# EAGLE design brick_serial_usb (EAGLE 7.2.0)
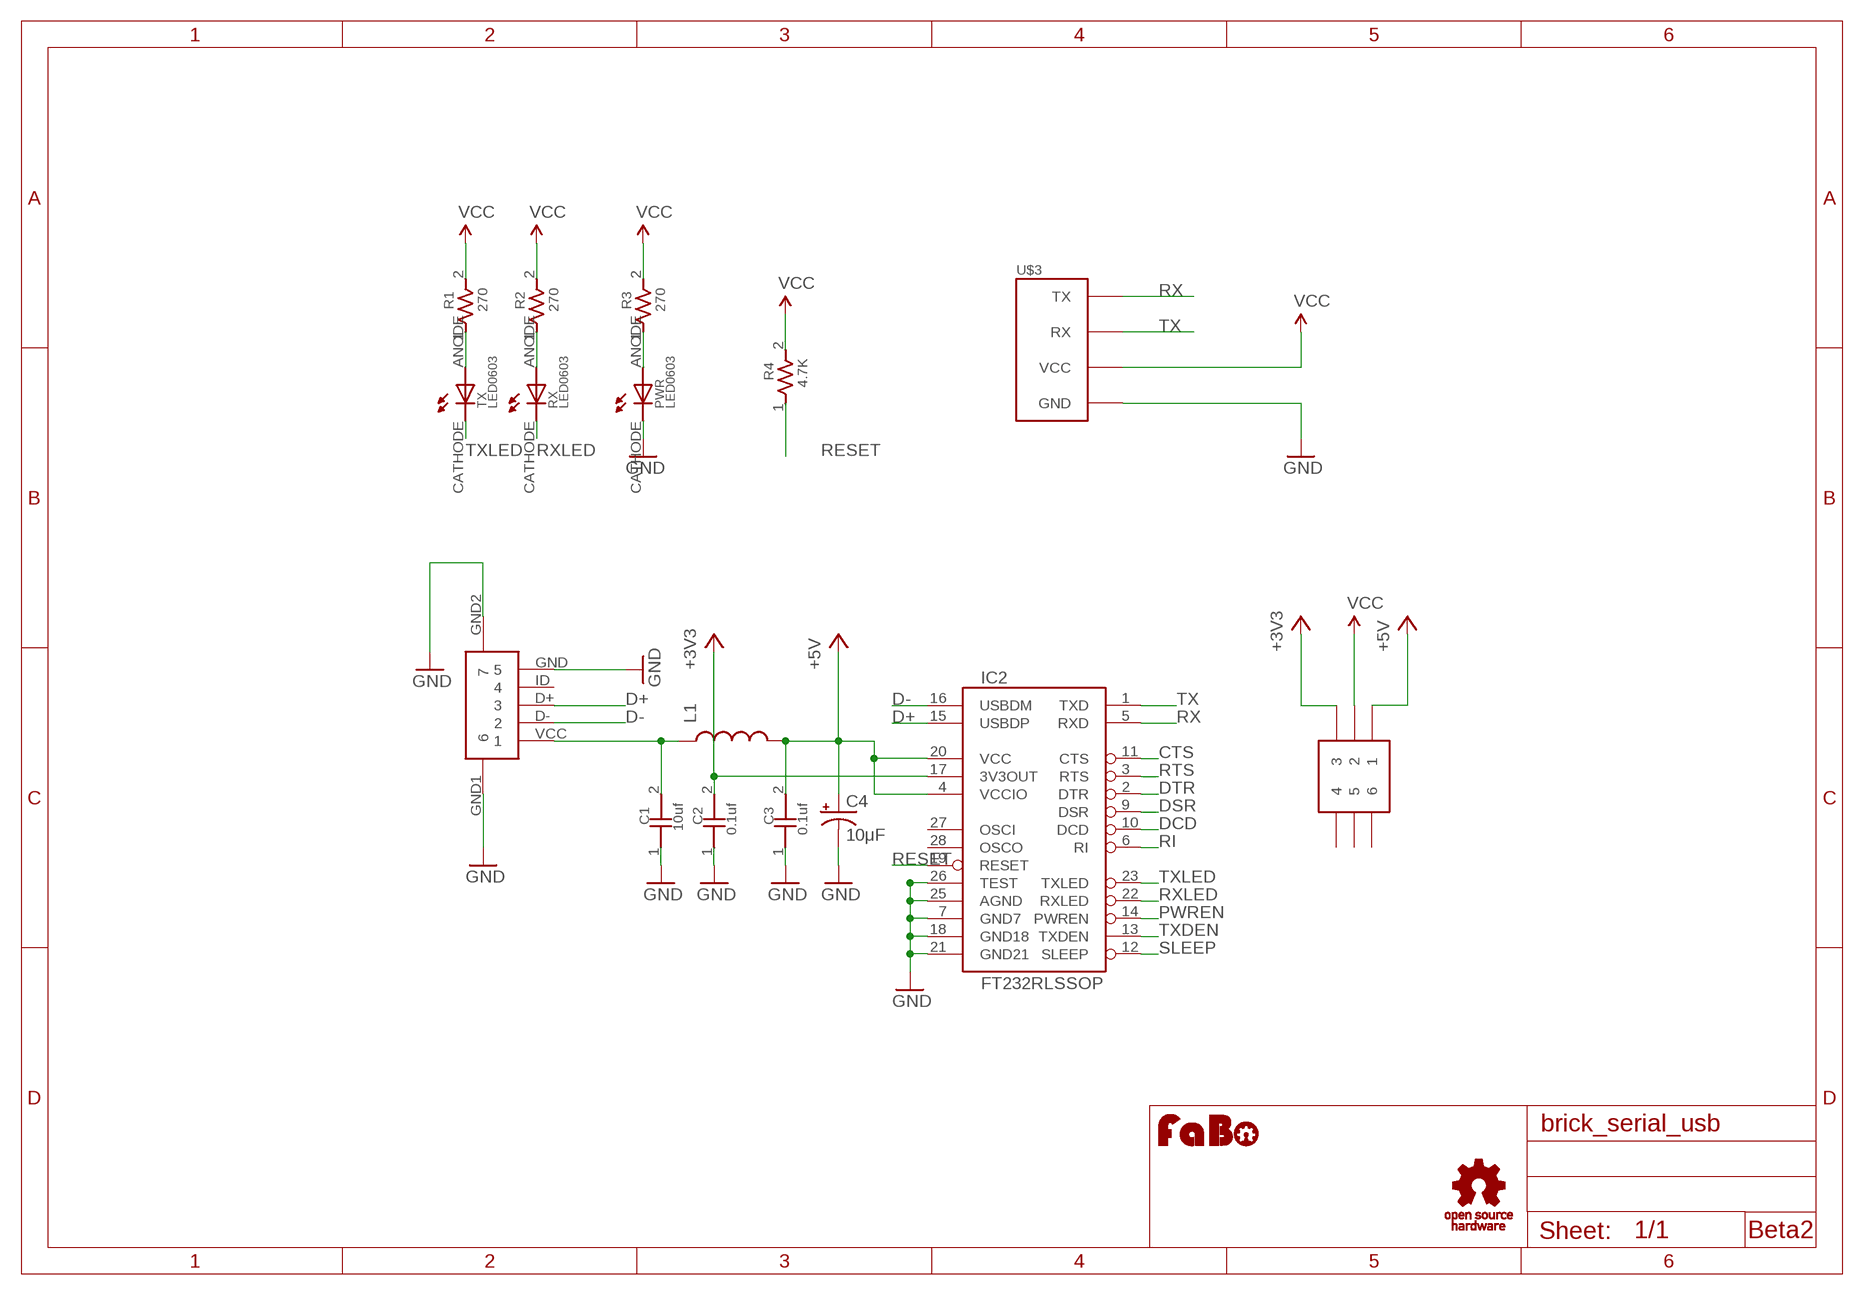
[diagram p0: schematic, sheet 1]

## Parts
C1  10uf  CAPACITOR0603  [0603]
C2  0.1uf  CAPACITOR0603  [0603]
C3  0.1uf  CAPACITOR0603  [0603]
C4  10μF  CAP_POL1206  [EIA3216]
IC2  FT232RLSSOP  [SSOP28DB]
L1  INDUCTOR0603  [0603]
PWR  LED0603  [0603]
R1  270  RESISTOR0603  [0603]
R2  270  RESISTOR0603  [0603]
R3  270  RESISTOR0603  [0603]
R4  4.7K  RESISTOR0603  [0603]
RX  LED0603  [0603]
TX  LED0603  [0603]
U$1  USB-MICRO-B-FEMALE  [USB-MICRO-B-FEMALE]
U$2  C&K_JS202011SCQN  [C&K_JS202011SCQN]
U$3  BRICK_SERIAL  [BRICK_SERIAL]
U$5  LOGO_OSHW_T-S  [LOGO_OSHW_T_S]
U$6  LOGO_FABO-S  [LOGO_FABO_S]

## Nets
+3V3: C2.2 IC2.17(3V3OUT) U$2.3
+5V: C3.2 C4.A(+) IC2.4(VCCIO) IC2.20(VCC) L1.2 U$2.1
CTS: IC2.11(CTS)
D+: IC2.15(USBDP) U$1.D+
D-: IC2.16(USBDM) U$1.D-
DCD: IC2.10(DCD)
DSR: IC2.9(DSR)
DTR: IC2.2(DTR)
GND: C1.1 C2.1 C3.1 C4.C(-) IC2.7(GND7) IC2.18(GND18) IC2.21(GND21) IC2.25(AGND) IC2.26(TEST) PWR.CATHODE U$1.GND U$1.GND1 U$1.GND2 U$3.GND
N$1: C1.2 L1.1 U$1.VCC
N$2: R1.1 TX.ANODE
N$5: R2.1 RX.ANODE
N$6: PWR.ANODE R3.1
PWREN: IC2.14(PWREN)
RESET: IC2.19(RESET) R4.1
RI: IC2.6(RI)
RTS: IC2.3(RTS)
RX: IC2.5(RXD) U$3.TX
RXLED: IC2.22(RXLED) RX.CATHODE
SLEEP: IC2.12(SLEEP)
TX: IC2.1(TXD) U$3.RX
TXDEN: IC2.13(TXDEN)
TXLED: IC2.23(TXLED) TX.CATHODE
VCC: R1.2 R2.2 R3.2 R4.2 U$2.2 U$3.VCC
Unconnected: IC2.27(OSCI) IC2.28(OSCO) U$1.ID U$2.4 U$2.5 U$2.6

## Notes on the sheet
- Beta2

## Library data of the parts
C1-C3 = GClue-Capacitor:CAPACITOR
C4 = SparkFun:CAP_POL: Capacitor Polarized
IC2 = SparkFun:FT232RL: USB UART FT232RL 4th Generation USB UART (USB <-> Serial) Controller. Spark Fun Electronics SKU : COM-00650
L1 = SparkFun:INDUCTOR: Inductors
PWR RX TX = GClue-LED:LED
R1-R4 = GClue-Resistors:RESISTOR
U$1 = gclue:USB-MICRO-B-FEMALE
U$2 = gclueParts:C&K_JS202011SCQN
U$3 = gclue:BRICK_SERIAL: FaBo Brick 4pin(SERIAL)
U$5 = gclue:LOGO_OSHW_T
U$6 = FaBo:LOGO_FABO

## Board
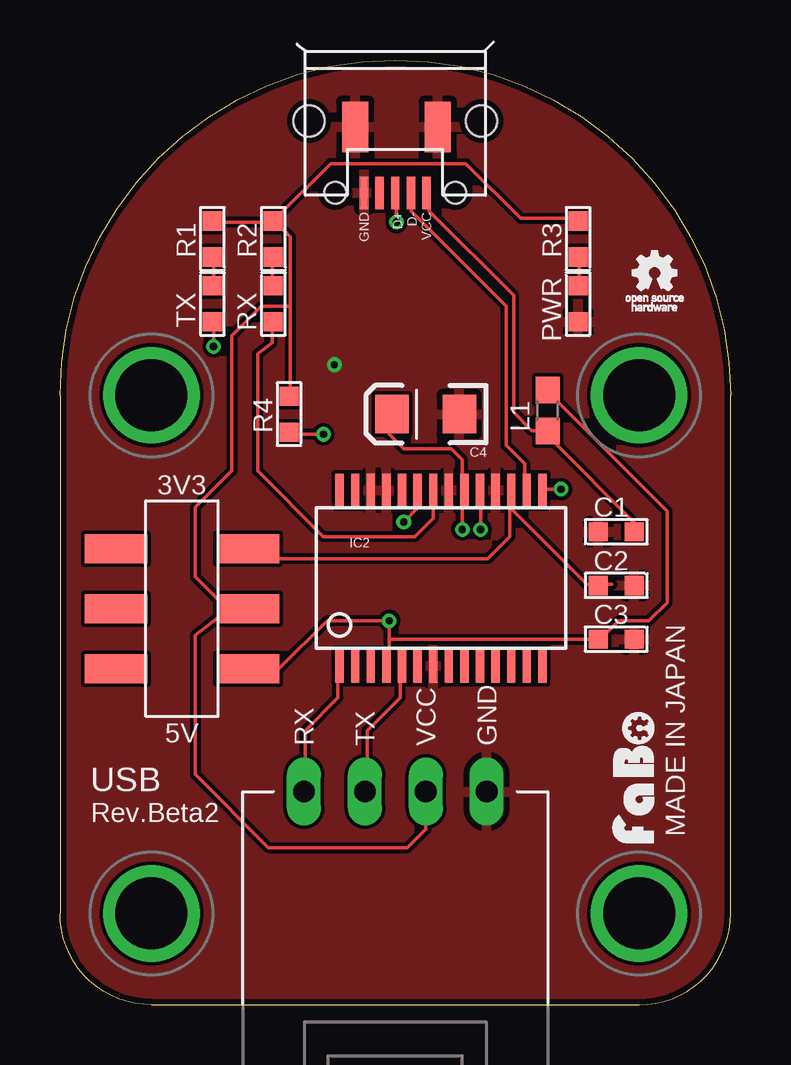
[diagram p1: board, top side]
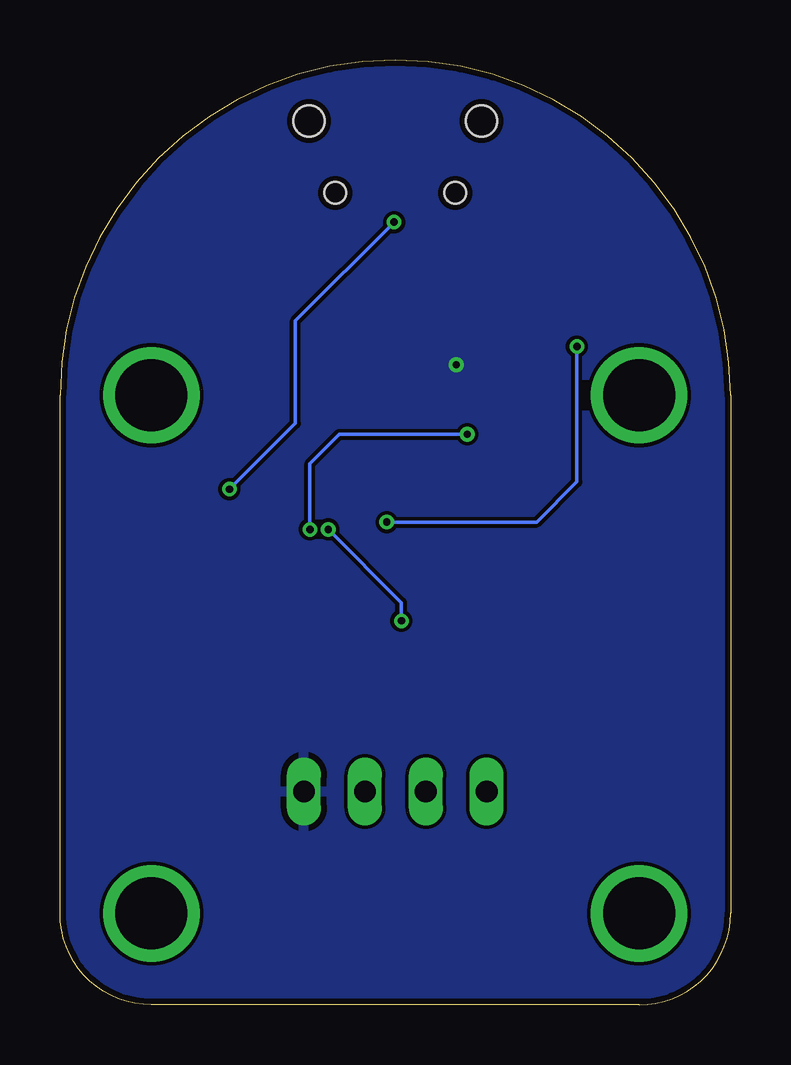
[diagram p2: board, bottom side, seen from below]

Size 27.94 x 39.37 mm. Coordinates in mm from the lower left corner, seen from the top.
Copper layers (1*16): Top 0.035mm / dielectric 1.5mm / Bottom 0.035mm
Design rules "Elecrow_2-layer_eagle_rule": minimum track width 6mil, minimum drill 12mil, track to track 6mil, track to pad 6mil, pad to pad 6mil, via to via 6mil, smd to smd 0mil, copper to edge 10mil, drill to drill 10mil, minimum pad ring 10mil, minimum via ring 6mil, stop-mask expansion 2mil, vias tented up to drill 100mil, thermal gap 10mil

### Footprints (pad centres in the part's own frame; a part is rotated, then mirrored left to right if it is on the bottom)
0603 = smd 0.8 x 0.8: 1 -0.75,0; 2 0.75,0
EIA3216 = smd 1.4 x 1.6: A 1.4,0; C -1.4,0
SSOP28DB = smd 0.348 x 1.397: 1 -4.225,-3.656; 2 -3.575,-3.656; 3 -2.925,-3.656; 4 -2.275,-3.656; 5 -1.625,-3.656; 6 -0.975,-3.656; 7 -0.325,-3.656; 8 0.325,-3.656; 9 0.975,-3.656; 10 1.625,-3.656; 11 2.275,-3.656; 12 2.925,-3.656; 13 3.575,-3.656; 14 4.225,-3.656; 15 4.225,3.656; 16 3.575,3.656; 17 2.925,3.656; 18 2.275,3.656; 19 1.625,3.656; 20 0.975,3.656; 21 0.325,3.656; 22 -0.325,3.656; 23 -0.975,3.656; 24 -1.625,3.656; 25 -2.275,3.656; 26 -2.925,3.656; 27 -3.575,3.656; 28 -4.225,3.656
0603' = smd 1.1 x 1: 1 -0.85,0; 2 0.85,0
0603'' = smd 0.8 x 0.8: ANODE -0.75,0; CATHODE 0.75,0
USB-MICRO-B-FEMALE = smd 1.35 x 0.35: D+ 3,0; D- 3,0.65; GND 3,-1.3; ID 3,-0.65; VCC 3,1.3 | smd 2.1 x 1.1: GND1 0.246,1.77; GND2 0.246,-1.67 | hole 1.3: 0,3.6; 0,-3.6 | hole 0.9: 3,2.5; 3,-2.5
C&K_JS202011SCQN = smd 2.6 x 1.2: 1 -2.75,2.5; 2 -2.75,0; 3 -2.75,-2.5; 4 2.75,-2.5; 5 2.75,0; 6 2.75,2.5
BRICK_SERIAL = drill 0.9 long: GND 3.81,-10.16; RX -3.81,-10.16; TX -1.27,-10.16; VCC 1.27,-10.16 | drill 3 pad 3.81: P$5 -10.16,6.35; P$6 10.16,6.35; P$7 -10.16,-15.24; P$8 10.16,-15.24

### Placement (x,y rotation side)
C1  23.18,19.71 0 top
C2  23.18,17.48 180 top
C3  23.18,15.24 180 top
C4  15.24,24.61 180 top
IC2  15.88,17.78 0 top
L1  [0603']  20.32,24.77 90 top
PWR  LED0603  [0603'']  21.59,29.21 270 top
R1  6.35,31.92 90 top
R2  8.89,31.92 90 top
R3  21.59,31.92 90 top
R4  9.55,24.61 90 top
RX  LED0603  [0603'']  8.89,29.21 270 top
TX  LED0603  [0603'']  6.35,29.21 270 top
U$1  13.97,36.83 270 top
U$2  5.08,16.51 180 top
U$3  13.97,19.05 0 top
U$5  24.77,30.48 0 top
U$6  24.77,9.53 90 top

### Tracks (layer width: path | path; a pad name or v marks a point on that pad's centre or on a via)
+3V3
  Top 0.152: 18.75,20.73 21.95,17.53 23,17.53 C2.2 | 18.75,20.73 18.75,20.88 IC2.17 | 18.75,20.73 18.75,19.51 17.83,18.59 8.99,18.59 U$2.3
+5V  (via drill 0.3)
  Top 0.152: v16.76,19.81 16.76,21.49 IC2.20 16.76,21.34 v16.76,19.81 | v16.76,19.81 16.76,22.71 16.31,23.16 14.33,23.16 13.72,23.77 13.72,24.69 C4.A | 13.72,15.24 C3.2 22.52,15.24 23.28,16 24.54,16 25.3,16.76 25.3,20.57 20.73,25.15 20.42,25.6 L1.2 | 13.72,15.24 13.72,14.17 IC2.4 | 13.72,15.24 v13.72,16 11.12,16 9.14,14.02 7.92,14.02 U$2.1
  Bottom 0.152: v16.76,19.81 13.72,16.76 v13.72,16
D+  (via drill 0.3)
  Top 0.152: 14.02,34.44 14.02,33.83 | v14.02,32.61 14.02,33.83 | v20.88,21.49 20.12,21.49 IC2.15 | 14.02,33.83 U$1.D+
  Bottom 0.152: v14.02,32.61 18.14,28.5 18.14,24.23 v20.88,21.49
D-
  Top 0.152: U$1.D- 14.63,33.68 14.63,33.07 18.59,29.11 18.59,23.32 19.36,22.55 19.36,21.64 IC2.16
GND  (via drill 0.3)
  other vias: 11.43,26.67
  pour Bottom: -1.27,-1.27 29.21,-1.27 29.21,40.64 -1.27,40.64
  pour Top: -1.27,-1.27 29.21,-1.27 29.21,40.64 -1.27,40.64
N$1
  Top 0.152: C1.2 23.89,19.81 24.21,19.81 20.27,23.77 L1.1 20.27,23.93 19.66,23.93 18.9,24.69 18.9,29.57 15.39,33.07 15.39,33.22 U$1.VCC
N$2
  Top 0.152: TX.ANODE 6.4,30.02 6.4,31.09 R1.1
N$5
  Top 0.152: RX.ANODE 8.84,30.02 8.84,31.09 R2.1
N$6
  Top 0.152: PWR.ANODE 21.64,30.02 21.64,31.09 R3.1
RESET  (via drill 0.3)
  Top 0.152: v10.97,23.77 9.6,23.77 R4.1 | v17.53,19.81 17.53,20.88 IC2.19
  Bottom 0.152: v17.53,19.81 17.53,22.55 16.31,23.77 v10.97,23.77
RX
  Top 0.152: U$3.TX 12.8,8.99 12.8,11.43 14.17,12.8 14.17,14.02 14.25,14.1 IC2.5
RXLED
  Top 0.152: RX.CATHODE 8.84,28.35 8.84,27.58 8.23,27.13 8.23,22.25 10.97,19.51 14.78,19.51 15.54,20.27 15.54,21.34 IC2.22
TX
  Top 0.152: IC2.1 11.58,14.02 11.58,12.8 10.21,11.43 10.21,8.99 U$3.RX
TXLED  (via drill 0.3)
  Top 0.152: v6.4,27.43 6.4,28.35 TX.CATHODE | v14.33,20.12 14.94,20.73 14.94,21.34 IC2.23
  Bottom 0.152: v14.33,20.12 8.08,20.12 6.4,21.79 v6.4,27.43
VCC
  Top 0.152: 9.6,29.11 9.6,25.6 R4.2 | 9.6,29.11 9.6,32 8.99,32.61 R2.2 | R1.2 6.4,32.61 8.84,32.61 R2.2 | R3.2 21.49,32.77 19.2,32.77 16.92,35.05 11.28,35.05 8.99,32.77 R2.2 | 7.01,16.46 5.64,17.83 5.64,20.73 7.16,22.25 7.16,27.89 8.38,29.11 9.6,29.11 | U$3.VCC 15.24,7.32 14.48,6.55 8.69,6.55 5.64,9.6 5.64,15.39 7.01,16.46 | 7.01,16.46 7.77,16.46 U$2.2

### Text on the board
tPlace: 3V3 | 5V | MADE IN JAPAN | USB | Rev.Beta2

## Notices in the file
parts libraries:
SparkFun: Licensing: CC v3.0 Share-Alike You are welcome to use this library for commercial purposes.
